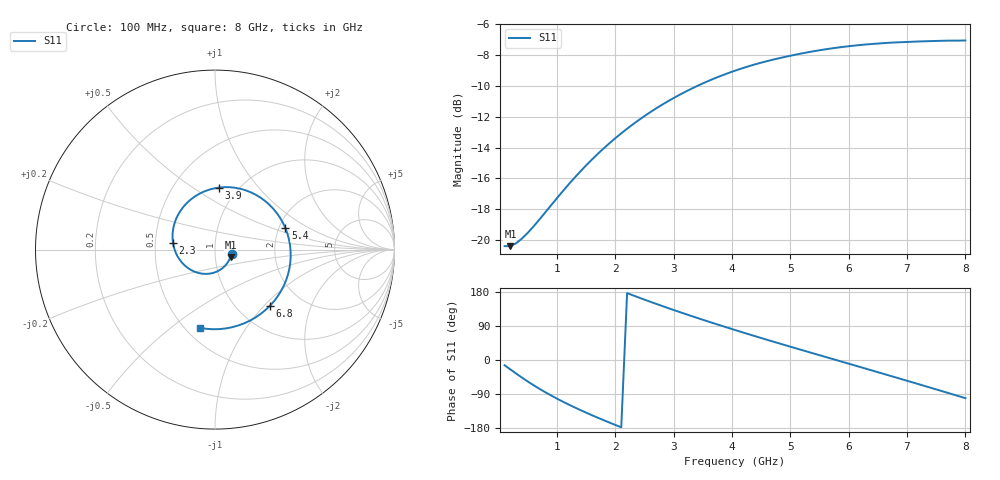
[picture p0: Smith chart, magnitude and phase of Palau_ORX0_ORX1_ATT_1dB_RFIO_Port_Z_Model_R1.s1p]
! Created Fri Oct  9 14:28:49 2020
! Palau ORX0/ORX1 RFIO Port Impedance Model.
! Attenuation  : 1 dB.
! Revision		: R1.
! Impedance Mode 	: Balanced Differential-Mode.
! Impedance Format 	: Series Equivalent Differential Impedance (SEDZ).
# hz S ma R 100
! 1 Port Network Data from SP1.SP block
! freq  magS11  angS11
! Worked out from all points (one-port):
!   80 points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, 100 MHz to 8 GHz, reference 100 ohm
!   lowest |S11| = -20.4 dB at 200 MHz (marker M1), VSWR 1.21, Z = 119 - j9.66 ohm
!   |S11| at or under -10 dB: start of sweep to 3.402 GHz
!   S11 on the Smith chart (normalised r, x): 100 MHz: 1.20, -0.06; 2.3 GHz: 0.62, +0.05; 3.9 GHz: 0.82, +0.64; 5.4 GHz: 2.16, +0.63; 6.8 GHz: 1.39, -1.08; 8 GHz: 0.59, -0.64
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1e8  0.09551 -13.9
2e8  0.09548 -25.0
4e8  0.1012 -46.7
7e8  0.1168 -76.3
1.1e9  0.1442 -110.0
1.3e9  0.1593 -125.0
1.6e9  0.1827 -145.9
1.8e9  0.1984 -158.9
2.1e9  0.222 -177.5
2.3e9  0.2375 170.7
2.7e9  0.2676 148.0
3.1e9  0.2961 126.6
3.5e9  0.3225 106.1
3.9e9  0.3463 86.4
4.1e9  0.3571 76.8
4.3e9  0.3672 67.3
4.6e9  0.3808 53.3
4.8e9  0.3889 44.2
5.1e9  0.4 30.6
5.4e9  0.41 17.1
5.8e9  0.4211 -0.8
6.1e9  0.4277 -14.2
6.4e9  0.4329 -27.7
6.8e9  0.4379 -45.7
7.1e9  0.4403 -59.3
7.4e9  0.4422 -73.0
7.6e9  0.4433 -82.2
8e9  0.4444 -100.7
